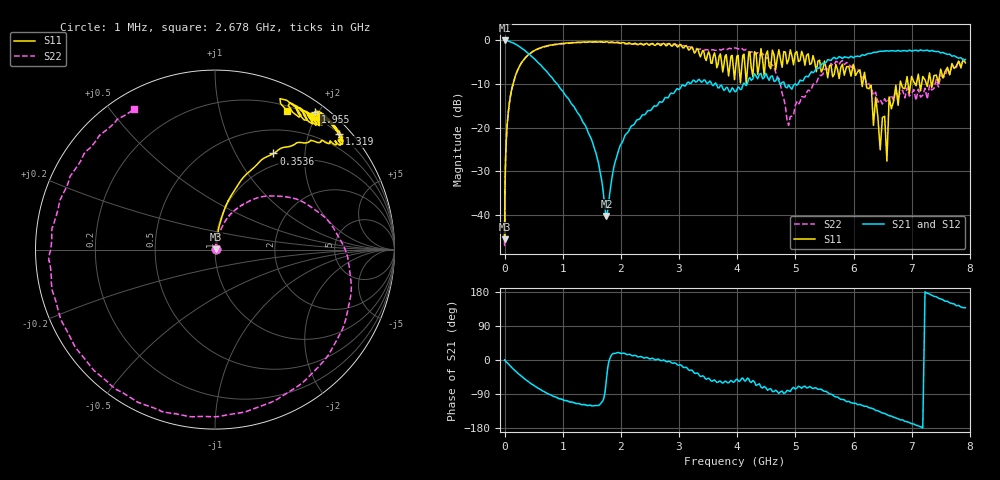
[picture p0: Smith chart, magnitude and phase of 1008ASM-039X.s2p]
!s-Parameter Generated by FASTRON Sdn. Bhd.
!FASTRON P/N : 1008ASM-039X
!Keysight Technologies: E5071C_MY46733604_B.14.02
!Date: Tue Nov 21 11:24:05 2023
!Version  :Rev00  Wed Nov 22 15:48:07 2023
!Data & Calibration Information:
!Freq  S11:SOLT2(ON)  S21:SOLT2(ON)  S12:SOLT2(ON)  S22:SOLT2(ON)
!PortZ  Port1:50+j0  Port2:50+j0
!When reading reference impedance value at option line is always used.
! Remarks : This data is being provided solely for informational purposes.
# Hz S dB R 50
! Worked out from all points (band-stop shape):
!   1599 points, 1 MHz to 7.923 GHz, reference 50 ohm
!   highest |S21| = -0.03 dB at 6.301 MHz (marker M1); lowest = -40.3 dB at 1.752 GHz (marker M2)
!   |S21| within 3 dB of the highest: start of sweep to 411.7 MHz; 6.261 GHz to 7.574 GHz (1.312 GHz wide, 19 % of centre)
!   lowest |S11| = -45.6 dB at 1.505 MHz (marker M3), VSWR 1.01, Z = 50.5 + j0.234 ohm
!   |S11| at or under -10 dB: start of sweep to 146 MHz; 6.217 GHz to 6.8 GHz (583.5 MHz wide, 8.96 % of centre); 6.821 GHz to 6.897 GHz (76 MHz wide, 1.11 % of centre)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
!   |S22| runs from -47.2 to -0.4 dB; largest |S21 - S12| = 0.014
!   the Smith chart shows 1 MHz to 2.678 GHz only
!   S11 on the Smith chart (normalised r, x): 1 MHz: 1.01, +0.00; 353.6 MHz: 0.82, +1.44; 1.319 GHz: 0.20, +2.53; 1.955 GHz: 0.12, +1.96; 2.678 GHz: 0.25, +1.62
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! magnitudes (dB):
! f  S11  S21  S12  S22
! 1 MHz  -43.4  0.0  -0.1  -43.5
! 1.505 MHz  -45.6  0.0  -0.1  -45.3
! 4.479 MHz  -38.0  -0.1  -0.1  -38.3
! 6.301 MHz  -35.4  0.0  -0.1  -37.6
! 19.95 MHz  -26.3  -0.1  -0.1  -26.1
! 89.01 MHz  -13.8  -0.3  -0.3  -13.9
! 353.6 MHz  -4.1  -2.4  -2.4  -4.1
! 398.5 MHz  -3.4  -2.9  -2.9  -3.5
! 809.2 MHz  -1.1  -8.4  -8.4  -1.2
! 1.319 GHz  -0.5  -17.9  -17.9  -0.5
! 1.543 GHz  -0.3  -24.7  -24.8  -0.4
! 1.752 GHz  -0.3  -40.3  -40.3  -0.5
! 1.784 GHz  -0.5  -37.7  -37.7  -0.5
! 1.955 GHz  -0.4  -25.5  -25.5  -0.7
! 2.678 GHz  -1.2  -14.1  -14.1  -0.9
! 4.325 GHz  -3.0  -8.2  -8.3  -3.0
! 4.968 GHz  -5.6  -10.3  -10.3  -17.2
! 5.752 GHz  -8.8  -3.7  -3.7  -5.5
! 6.034 GHz  -8.1  -3.7  -3.7  -7.0
! 6.496 GHz  -17.7  -2.5  -2.5  -14.6
! 7.229 GHz  -9.1  -2.3  -2.3  -11.0
! 7.923 GHz  -5.2  -4.4  -4.4  -4.6
